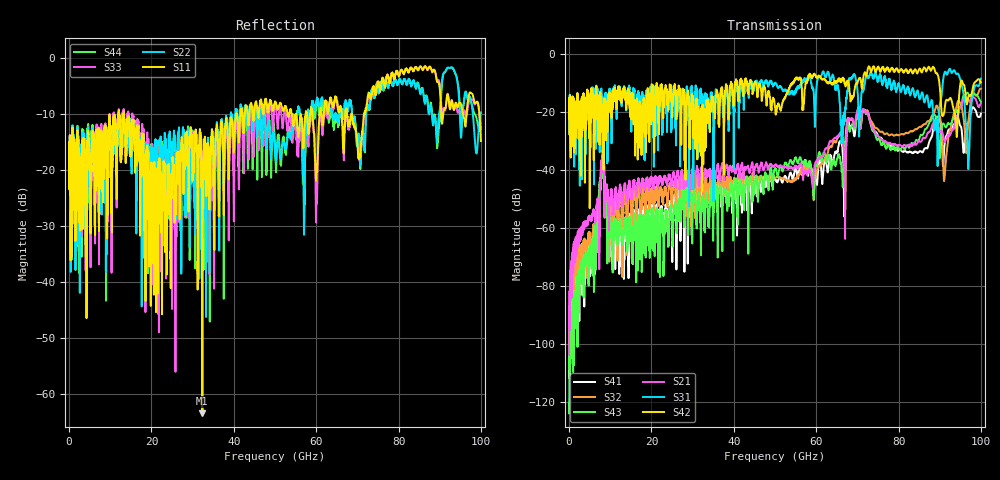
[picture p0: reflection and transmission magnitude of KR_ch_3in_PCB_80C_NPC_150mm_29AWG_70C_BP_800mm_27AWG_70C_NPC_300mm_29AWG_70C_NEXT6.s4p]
# GHz S RI R 45
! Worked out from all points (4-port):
!   4000 points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, 25 MHz to 100 GHz, reference 45 ohm
!   strongest paths, dB at 25 MHz, 25.02 GHz, 50.02 GHz, 75.03 GHz, 100 GHz:
!     S42: -20.7, -17.7, -18.0, -4.4, -9.7
!     S31: -20.7, -20.8, -10.2, -8.7, -8.4
!     S21: -103.9, -43.6, -38.1, -28.3, -17.0
!     S43: -124.1, -58.9, -39.3, -29.4, -16.4
!     S32: -108.7, -52.0, -42.7, -25.9, -11.9
!     S41: -111.9, -69.1, -43.0, -28.1, -20.5
!   lowest |S11| = -63.4 dB at 32.38 GHz (marker M1), VSWR 1.00, Z = 45.1 + j0.0134 ohm
!   |S11| at or under -10 dB: start of sweep to 12.06 GHz; 13.32 GHz to 40.54 GHz (27.22 GHz wide, 101 % of centre); 68.65 GHz to 71.57 GHz (2.922 GHz wide, 4.17 % of centre)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
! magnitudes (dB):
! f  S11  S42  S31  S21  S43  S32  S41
! 25 MHz  -16.6  -20.7  -20.7  -103.9  -124.1  -108.7  -111.9
! 8.025 GHz  -23.7  -25.3  -21.0  -41.0  -37.9  -39.5  -38.4
! 11.7 GHz  -14.2  -12.9  -13.9  -53.5  -61.0  -58.3  -61.8
! 32.38 GHz  -63.4  -23.4  -21.9  -41.8  -49.2  -42.7  -44.6
! 91.25 GHz  -9.0  -18.3  -6.1  -30.2  -24.8  -41.2  -30.2
! 96.85 GHz  -7.7  -15.3  -36.0  -15.2  -13.4  -24.4  -23.8
! 100 GHz  -14.8  -9.7  -8.4  -17.0  -16.4  -11.9  -20.5
